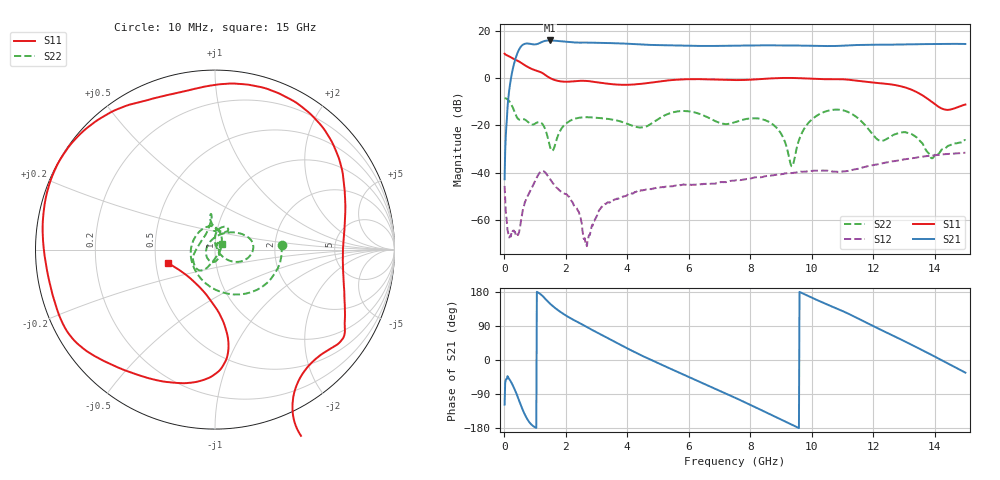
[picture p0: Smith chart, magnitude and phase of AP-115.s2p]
! MARKI MICROWAVE INC.
! Email:  info@markimicrowave.com  Phone:  408-778-4200
! Model Number:  AP-115  Date:  03/13
! Filename:		AP-115.S2P  Version: 1.0
! Description:  2-port S-parameter data for amplifier AP-115 measured at -20 dBm input power
! Frequency Measured: 	10 MHz to 15 GHz
! Measurements:		S11, S21, S12, S22
# Hz S  dB  R 50
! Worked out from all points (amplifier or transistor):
!   801 points, 10 MHz to 15 GHz, reference 50 ohm
!   highest |S21| = 15.8 dB at 1.472 GHz (marker M1)
!   |S21| within 3 dB of that: 517.7 MHz to end of sweep
!   unconditionally stable (mu >= 1): 1.533 GHz to 8.457 GHz; 10.05 GHz to end of sweep
!   at 2.502 GHz: K = 23.70, MAG = 21.0 dB, |S12| = -60.7 dB
!   at 7.505 GHz: K = 2.84, MAG = 21.0 dB, |S12| = -43.3 dB
!   at 15 GHz: K = 3.45, MAG = 14.7 dB, |S12| = -31.6 dB
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1e7  10.22 -1.9  -42.81 -117.8  -45.61 3.7  -8.55 4.0
1.786375e8  8.95 -19.2  -3.37 -52.4  -66.93 41.1  -10.10 -49.2
3.285375e8  7.85 -29.2  6.53 -76.0  -65.08 -97.0  -14.22 -105.8
5.533875e8  6.31 -42.2  13.40 -122.4  -59.23 -8.2  -17.54 130.8
6.8455e8  5.20 -47.4  14.44 -146.7  -52.12 -68.5  -17.73 94.0
7.96975e8  4.37 -50.5  14.47 -162.2  -48.97 -96.0  -18.95 84.8
1.28415e9  1.68 -64.2  15.47 165.7  -39.48 139.7  -20.33 72.0
1.471525e9  0.04 -64.5  15.80 150.0  -42.41 92.2  -28.29 24.3
1.902488e9  -1.58 -51.9  15.38 122.7  -48.46 49.3  -20.64 -109.4
2.520825e9  -1.24 -35.5  14.88 94.4  -61.27 -16.0  -16.73 -128.4
3.139162e9  -2.08 -23.2  14.77 67.2  -55.06 111.2  -17.01 -145.8
3.83245e9  -2.93 -4.0  14.51 37.6  -50.39 75.4  -18.62 -169.8
5.012912e9  -1.55 32.2  13.83 -8.5  -46.24 24.1  -17.32 102.9
6.3058e9  -0.52 73.6  13.49 -55.8  -45.06 -23.7  -15.01 98.7
7.505e9  -0.93 102.4  13.59 -99.4  -43.29 -63.8  -18.70 58.6
8.872838e9  -0.10 138.7  13.73 -152.1  -40.90 -119.2  -21.30 87.9
9.360012e9  -0.04 154.8  13.68 -171.0  -40.19 -140.9  -37.37 23.4
1.001582e10  -0.38 178.4  13.55 164.0  -39.26 -171.0  -17.43 -30.7
1.149609e10  -1.24 -133.0  13.88 110.1  -38.39 139.3  -16.92 42.3
1.250791e10  -2.62 -97.0  14.02 69.6  -35.54 102.1  -25.28 -155.9
1.389449e10  -10.00 -90.2  14.31 13.6  -32.77 47.0  -33.87 -6.1
1.5e10  -11.25 -164.3  14.31 -33.4  -31.61 4.5  -26.47 38.5
